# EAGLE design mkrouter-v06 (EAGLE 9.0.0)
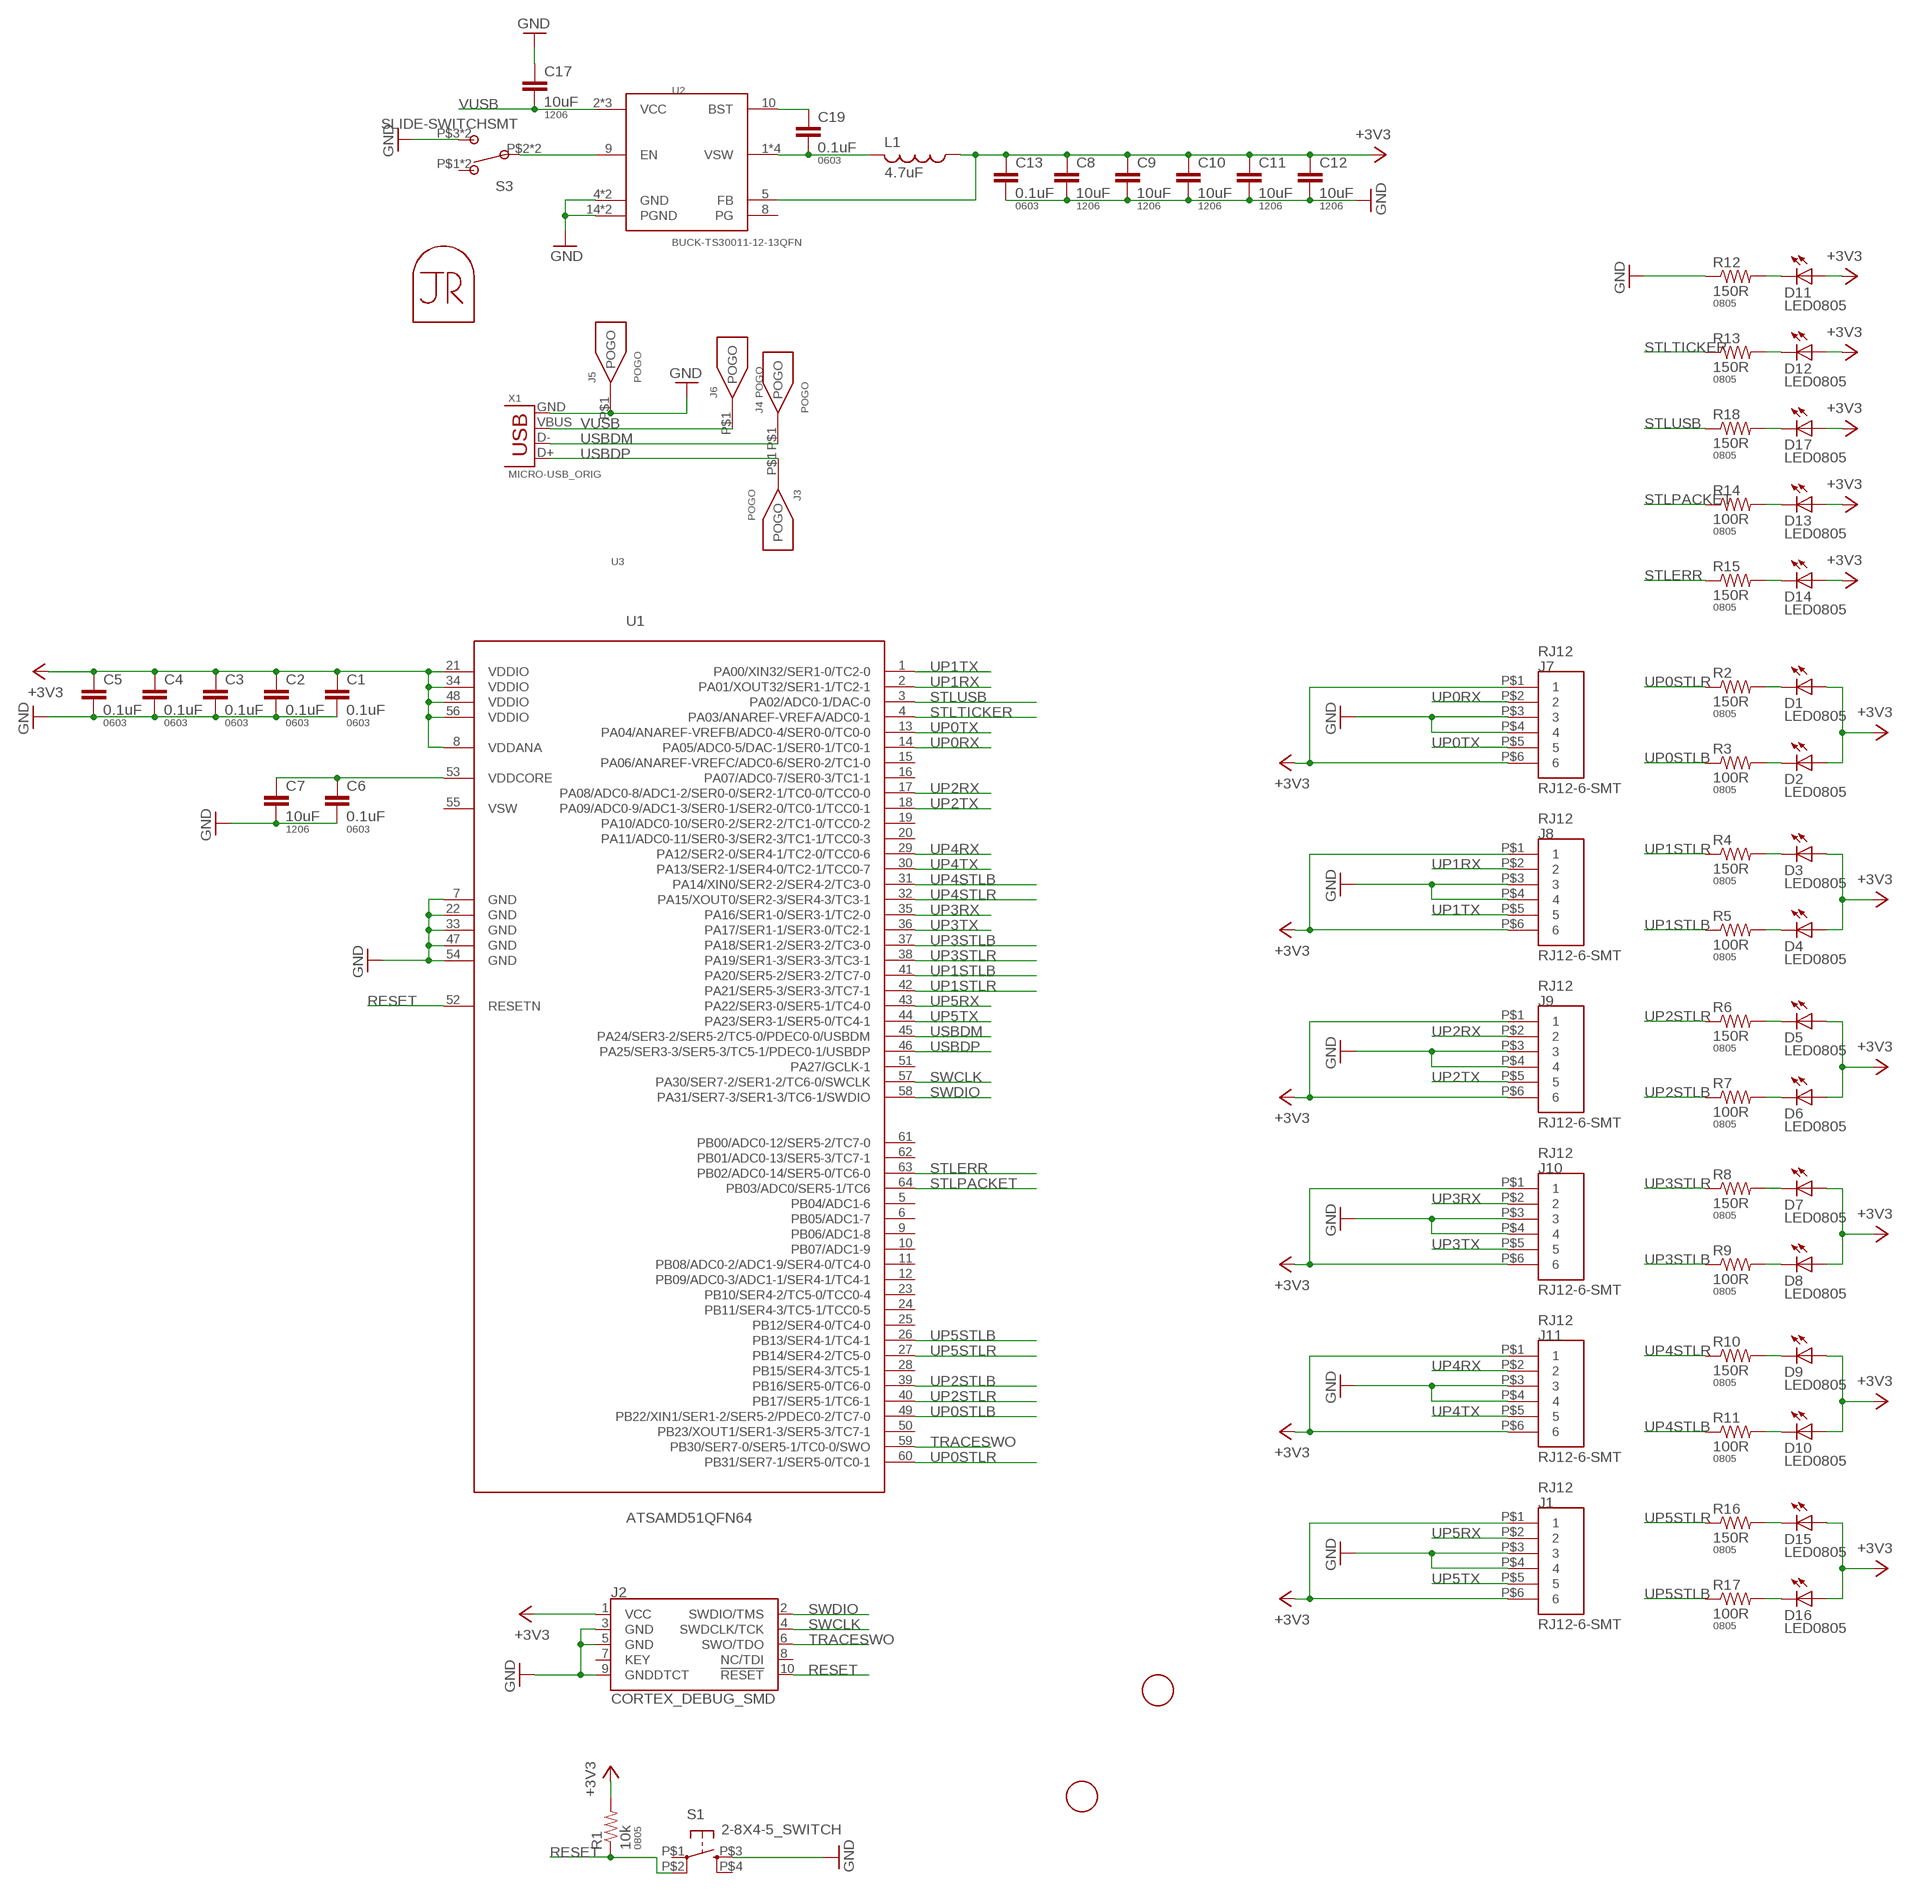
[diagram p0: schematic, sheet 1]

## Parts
C1  0.1uF  CAP0603-CAP  [0603-CAP]
C2  0.1uF  CAP0603-CAP  [0603-CAP]
C3  0.1uF  CAP0603-CAP  [0603-CAP]
C4  0.1uF  CAP0603-CAP  [0603-CAP]
C5  0.1uF  CAP0603-CAP  [0603-CAP]
C6  0.1uF  CAP0603-CAP  [0603-CAP]
C7  10uF  CAP1206  [1206]
C8  10uF  CAP1206  [1206]
C9  10uF  CAP1206  [1206]
C10  10uF  CAP1206  [1206]
C11  10uF  CAP1206  [1206]
C12  10uF  CAP1206  [1206]
C13  0.1uF  CAP0603-CAP  [0603-CAP]
C17  10uF  CAP1206  [1206]
C19  0.1uF  CAP0603-CAP  [0603-CAP]
D1  LED0805  [LED0805]
D2  LED0805  [LED0805]
D3  LED0805  [LED0805]
D4  LED0805  [LED0805]
D5  LED0805  [LED0805]
D6  LED0805  [LED0805]
D7  LED0805  [LED0805]
D8  LED0805  [LED0805]
D9  LED0805  [LED0805]
D10  LED0805  [LED0805]
D11  LED0805  [LED0805]
D12  LED0805  [LED0805]
D13  LED0805  [LED0805]
D14  LED0805  [LED0805]
D15  LED0805  [LED0805]
D16  LED0805  [LED0805]
D17  LED0805  [LED0805]
J1  RJ12-6-SMT  [RJ12-6-SMT]
J2  CORTEX_DEBUG_SMD  [SAMTECH_FTSH-105-01]
J3  POGO  [POGO]
J4  POGO  [POGO]
J5  POGO  [POGO]
J6  POGO  [POGO]
J7  RJ12-6-SMT  [RJ12-6-SMT]
J8  RJ12-6-SMT  [RJ12-6-SMT]
J9  RJ12-6-SMT  [RJ12-6-SMT]
J10  RJ12-6-SMT  [RJ12-6-SMT]
J11  RJ12-6-SMT  [RJ12-6-SMT]
L1  4.7uF  INDUCTOR  [NRS5020T4R7MMGJ]
MP1  JRTOMBSTONE  [JRTOMBSTONE]
R1  10k  RESISTOR0805-RES  [0805]
R2  150R  RESISTOR0805-RES  [0805]
R3  100R  RESISTOR0805-RES  [0805]
R4  150R  RESISTOR0805-RES  [0805]
R5  100R  RESISTOR0805-RES  [0805]
R6  150R  RESISTOR0805-RES  [0805]
R7  100R  RESISTOR0805-RES  [0805]
R8  150R  RESISTOR0805-RES  [0805]
R9  100R  RESISTOR0805-RES  [0805]
R10  150R  RESISTOR0805-RES  [0805]
R11  100R  RESISTOR0805-RES  [0805]
R12  150R  RESISTOR0805-RES  [0805]
R13  150R  RESISTOR0805-RES  [0805]
R14  100R  RESISTOR0805-RES  [0805]
R15  150R  RESISTOR0805-RES  [0805]
R16  150R  RESISTOR0805-RES  [0805]
R17  100R  RESISTOR0805-RES  [0805]
R18  150R  RESISTOR0805-RES  [0805]
S1  2-8X4-5_SWITCH  [TACT-SWITCH-KMR6]
S3  SLIDE-SWITCHSMT  [SLIDESWITCH-CL-SB-22A]
U1  ATSAMD51QFN64  [QFN-64-9X9MM]
U2  BUCK-TS30011-12-13QFN  [QFN16-3X3-TI-RTE]
U3  RASPBERRYPI-3BPLUS  [RASPBERRYPI-3BPLUS]
U$3  FIDUCIAL  [FIDUCIAL_1MM]
U$4  FIDUCIAL  [FIDUCIAL_1MM]
X1  MICRO-USB_ORIG  [DX4R005HJ5]

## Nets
+3V3: C1.1 C2.1 C3.1 C4.1 C5.1 C8.1 C9.1 C10.1 C11.1 C12.1 C13.1 D1.1(A) D2.1(A) D3.1(A) D4.1(A) D5.1(A) D6.1(A) D7.1(A) D8.1(A) D9.1(A) D10.1(A) D11.1(A) D12.1(A) D13.1(A) D14.1(A) D15.1(A) D16.1(A) D17.1(A) J1.P$1 J1.P$6 J2.1(VCC) J7.P$1 J7.P$6 J8.P$1 J8.P$6 J9.P$1 J9.P$6 J10.P$1 J10.P$6 J11.P$1 J11.P$6 L1.1 R1.2 U1.8(VDDANA) U1.21(VDDIO) U1.34(VDDIO) U1.48(VDDIO) U1.56(VDDIO) U2.5(FB)
BST: C19.1 U2.10(BST)
GND: C1.2 C2.2 C3.2 C4.2 C5.2 C6.2 C7.2 C8.2 C9.2 C10.2 C11.2 C12.2 C13.2 C17.1 J1.P$3 J1.P$4 J2.3(GND) J2.5(GND) J2.9(GNDDTCT) J5.P$1(POGO) J7.P$3 J7.P$4 J8.P$3 J8.P$4 J9.P$3 J9.P$4 J10.P$3 J10.P$4 J11.P$3 J11.P$4 R12.1 S1.P$3(S) S3.P$3 S3.P$6 U1.7(GND) U1.22(GND) U1.33(GND) U1.47(GND) U1.54(GND) U2.4(GND) U2.14(PGND) U2.15(PGND) U2.TH(GND) X1.GND
N$1: S3.P$2 S3.P$5 U2.9(EN)
N$2: D4.2(C) R5.2
N$3: D16.2(C) R17.2
N$4: D17.2(C) R18.2
N$5: D15.2(C) R16.2
N$6: D2.2(C) R3.2
N$8: D1.2(C) R2.2
N$9: D3.2(C) R4.2
N$10: D6.2(C) R7.2
N$11: D5.2(C) R6.2
N$12: D8.2(C) R9.2
N$13: D7.2(C) R8.2
N$14: D10.2(C) R11.2
N$15: D9.2(C) R10.2
N$16: D13.2(C) R14.2
N$17: D14.2(C) R15.2
N$22: D12.2(C) R13.2
N$23: D11.2(C) R12.2
RESET: J2.10(!RESET) R1.1 S1.P$2(P1) U1.52(RESETN)
STLERR: R15.1 U1.63(PB02/ADC0-14/SER5-0/TC6-0)
STLPACKET: R14.1 U1.64(PB03/ADC0/SER5-1/TC6)
STLTICKER: R13.1 U1.4(PA03/ANAREF-VREFA/ADC0-1)
STLUSB: R18.1 U1.3(PA02/ADC0-1/DAC-0)
SWCLK: J2.4(SWDCLK/TCK) U1.57(PA30/SER7-2/SER1-2/TC6-0/SWCLK)
SWDIO: J2.2(SWDIO/TMS) U1.58(PA31/SER7-3/SER1-3/TC6-1/SWDIO)
TRACESWO: J2.6(SWO/TDO) U1.59(PB30/SER7-0/SER5-1/TC0-0/SWO)
UP0RX: J7.P$2 U1.14(PA05/ADC0-5/DAC-1/SER0-1/TC0-1)
UP0STLB: R3.1 U1.49(PB22/XIN1/SER1-2/SER5-2/PDEC0-2/TC7-0)
UP0STLR: R2.1 U1.60(PB31/SER7-1/SER5-0/TC0-1)
UP0TX: J7.P$5 U1.13(PA04/ANAREF-VREFB/ADC0-4/SER0-0/TC0-0)
UP1RX: J8.P$2 U1.2(PA01/XOUT32/SER1-1/TC2-1)
UP1STLB: R5.1 U1.41(PA20/SER5-2/SER3-2/TC7-0)
UP1STLR: R4.1 U1.42(PA21/SER5-3/SER3-3/TC7-1)
UP1TX: J8.P$5 U1.1(PA00/XIN32/SER1-0/TC2-0)
UP2RX: J9.P$2 U1.17(PA08/ADC0-8/ADC1-2/SER0-0/SER2-1/TC0-0/TCC0-0)
UP2STLB: R7.1 U1.39(PB16/SER5-0/TC6-0)
UP2STLR: R6.1 U1.40(PB17/SER5-1/TC6-1)
UP2TX: J9.P$5 U1.18(PA09/ADC0-9/ADC1-3/SER0-1/SER2-0/TC0-1/TCC0-1)
UP3RX: J10.P$2 U1.35(PA16/SER1-0/SER3-1/TC2-0)
UP3STLB: R9.1 U1.37(PA18/SER1-2/SER3-2/TC3-0)
UP3STLR: R8.1 U1.38(PA19/SER1-3/SER3-3/TC3-1)
UP3TX: J10.P$5 U1.36(PA17/SER1-1/SER3-0/TC2-1)
UP4RX: J11.P$2 U1.29(PA12/SER2-0/SER4-1/TC2-0/TCC0-6)
UP4STLB: R11.1 U1.31(PA14/XIN0/SER2-2/SER4-2/TC3-0)
UP4STLR: R10.1 U1.32(PA15/XOUT0/SER2-3/SER4-3/TC3-1)
UP4TX: J11.P$5 U1.30(PA13/SER2-1/SER4-0/TC2-1/TCC0-7)
UP5RX: J1.P$2 U1.43(PA22/SER3-0/SER5-1/TC4-0)
UP5STLB: R17.1 U1.26(PB13/SER4-1/TC4-1)
UP5STLR: R16.1 U1.27(PB14/SER4-2/TC5-0)
UP5TX: J1.P$5 U1.44(PA23/SER3-1/SER5-0/TC4-1)
USBDM: J4.P$1(POGO) U1.45(PA24/SER3-2/SER5-2/TC5-0/PDEC0-0/USBDM) X1.D-
USBDP: J3.P$1(POGO) U1.46(PA25/SER3-3/SER5-3/TC5-1/PDEC0-1/USBDP) X1.D+
VDDCORE: C6.1 C7.1 U1.53(VDDCORE)
VSW: C19.2 L1.2 U2.1(VSW) U2.12(VSW) U2.13(VSW) U2.16(VSW)
VUSB: C17.2 J6.P$1(POGO) U2.2(VCC) U2.3(VCC) U2.11(VCC) X1.VBUS
Unconnected: J2.7(KEY) J2.8(NC/TDI) S1.P$1(P) S1.P$4(S1) S3.P$1 S3.P$4 U1.5(PB04/ADC1-6) U1.6(PB05/ADC1-7) U1.9(PB06/ADC1-8) U1.10(PB07/ADC1-9) U1.11(PB08/ADC0-2/ADC1-9/SER4-0/TC4-0) U1.12(PB09/ADC0-3/ADC1-1/SER4-1/TC4-1) U1.15(PA06/ANAREF-VREFC/ADC0-6/SER0-2/TC1-0) U1.16(PA07/ADC0-7/SER0-3/TC1-1) U1.19(PA10/ADC0-10/SER0-2/SER2-2/TC1-0/TCC0-2) U1.20(PA11/ADC0-11/SER0-3/SER2-3/TC1-1/TCC0-3) U1.23(PB10/SER4-2/TC5-0/TCC0-4) U1.24(PB11/SER4-3/TC5-1/TCC0-5) U1.25(PB12/SER4-0/TC4-0) U1.28(PB15/SER4-3/TC5-1) U1.50(PB23/XOUT1/SER1-3/SER5-3/TC7-1) U1.51(PA27/GCLK-1) U1.55(VSW) U1.61(PB00/ADC0-12/SER5-2/TC7-0) U1.62(PB01/ADC0-13/SER5-3/TC7-1) U2.8(PG)

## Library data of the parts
C1-C6 C13 C19 = borkedlabs-passives:CAP: Capacitor; PACKAGE: 0603
C7-C12 C17 = borkedlabs-passives:CAP: Capacitor; PACKAGE: 1206
D1-D17 = lights:LED: LED
J1 J7-J11 = connector:RJ12-6-SMT
J2 = SparkFun-Connectors:CORTEX_DEBUG: Cortex Debug Connector - 10 pin Supports JTAG debug, Serial Wire debug, and Serial Wire Viewer. PTH and SMD connector options available. General Connector Information Products: PTH Connector -via Digi-Key SparkFun PSoc SparkFun T
J3-J6 = connector:POGO
L1 = power:INDUCTOR
MP1 = connector:JRTOMBSTONE
R1-R18 = borkedlabs-passives:RESISTOR: Resistor; PACKAGE: 0805
S1 = fab:2-8X4-5_SWITCH
S3 = fab:SLIDE-SWITCH: SMD slide-switch AYZ0102AGRLC as found in the fablab inventory. Includes the mounting holes. Made by Zaerc.
U1 = microcontrollers:ATSAMD51
U2 = power:BUCK-TS30011-12-13
U3 = connector:RASPBERRYPI-3BPLUS
U$3 U$4 = borkedlabs-misc:FIDUCIAL: For use by pick and place machines to calibrate the vision/machine, 1mm
X1 = fab:MICRO-USB: SMD micro USB connector as found in the fablab inventory. Three footprint variants included: original, as described by manufacturer's datasheet for milling with the 1/100" bit for milling with the 1/64" bit Made by Zaerc.

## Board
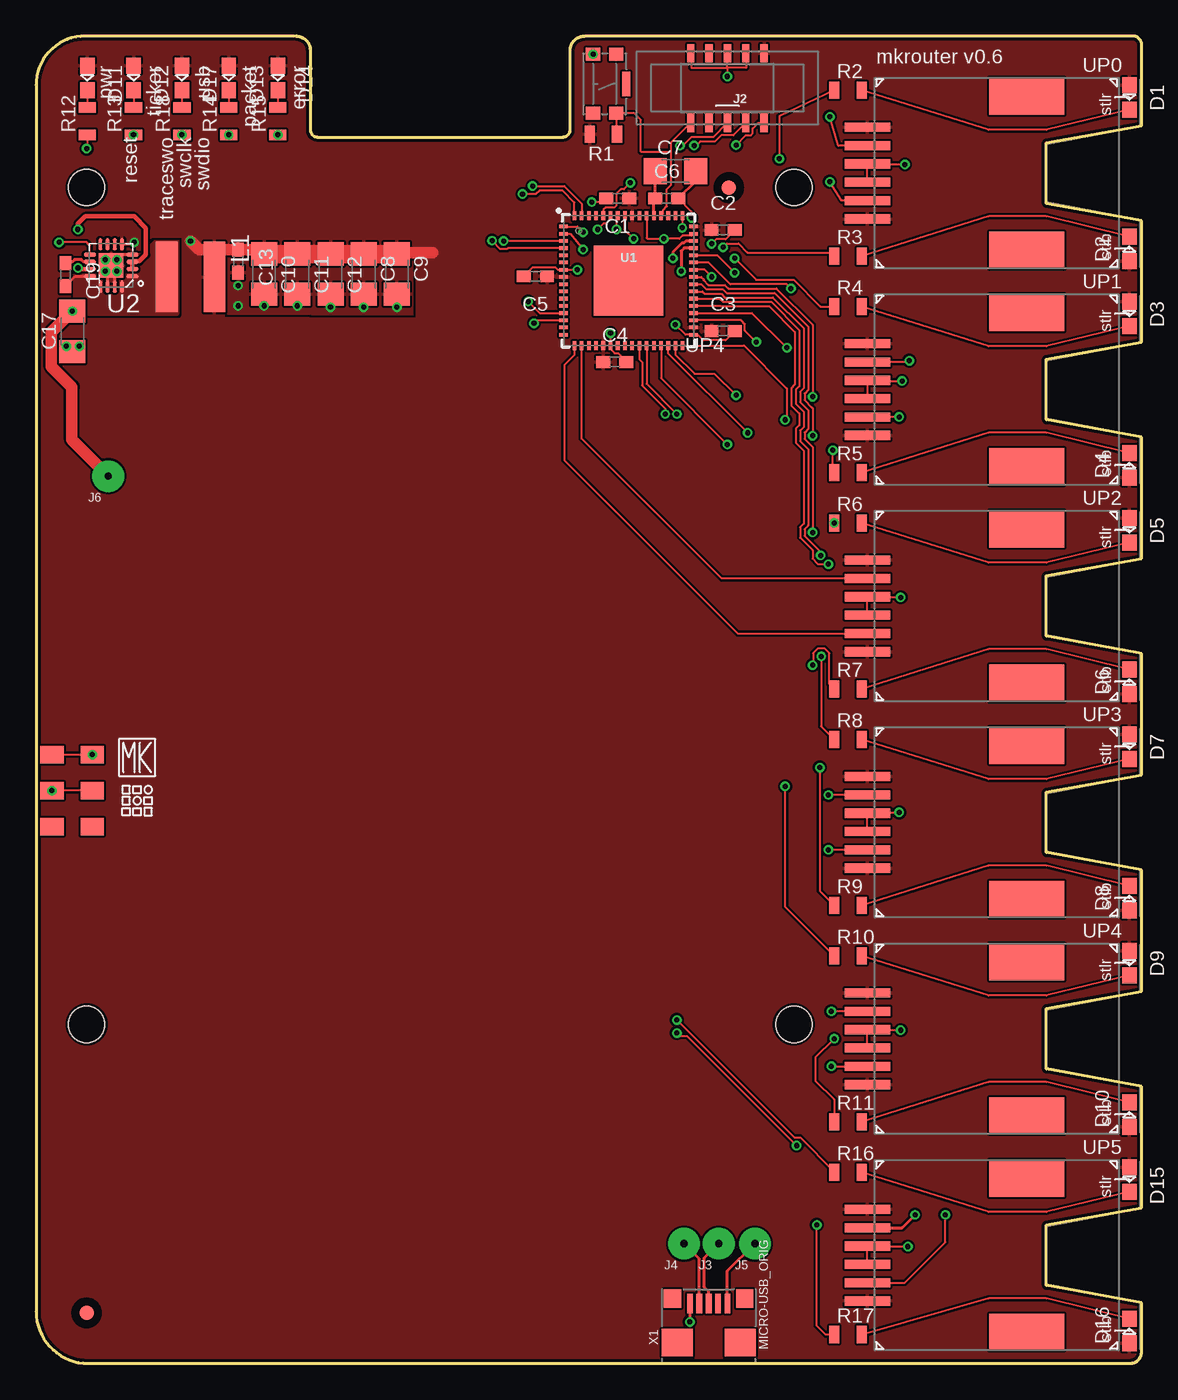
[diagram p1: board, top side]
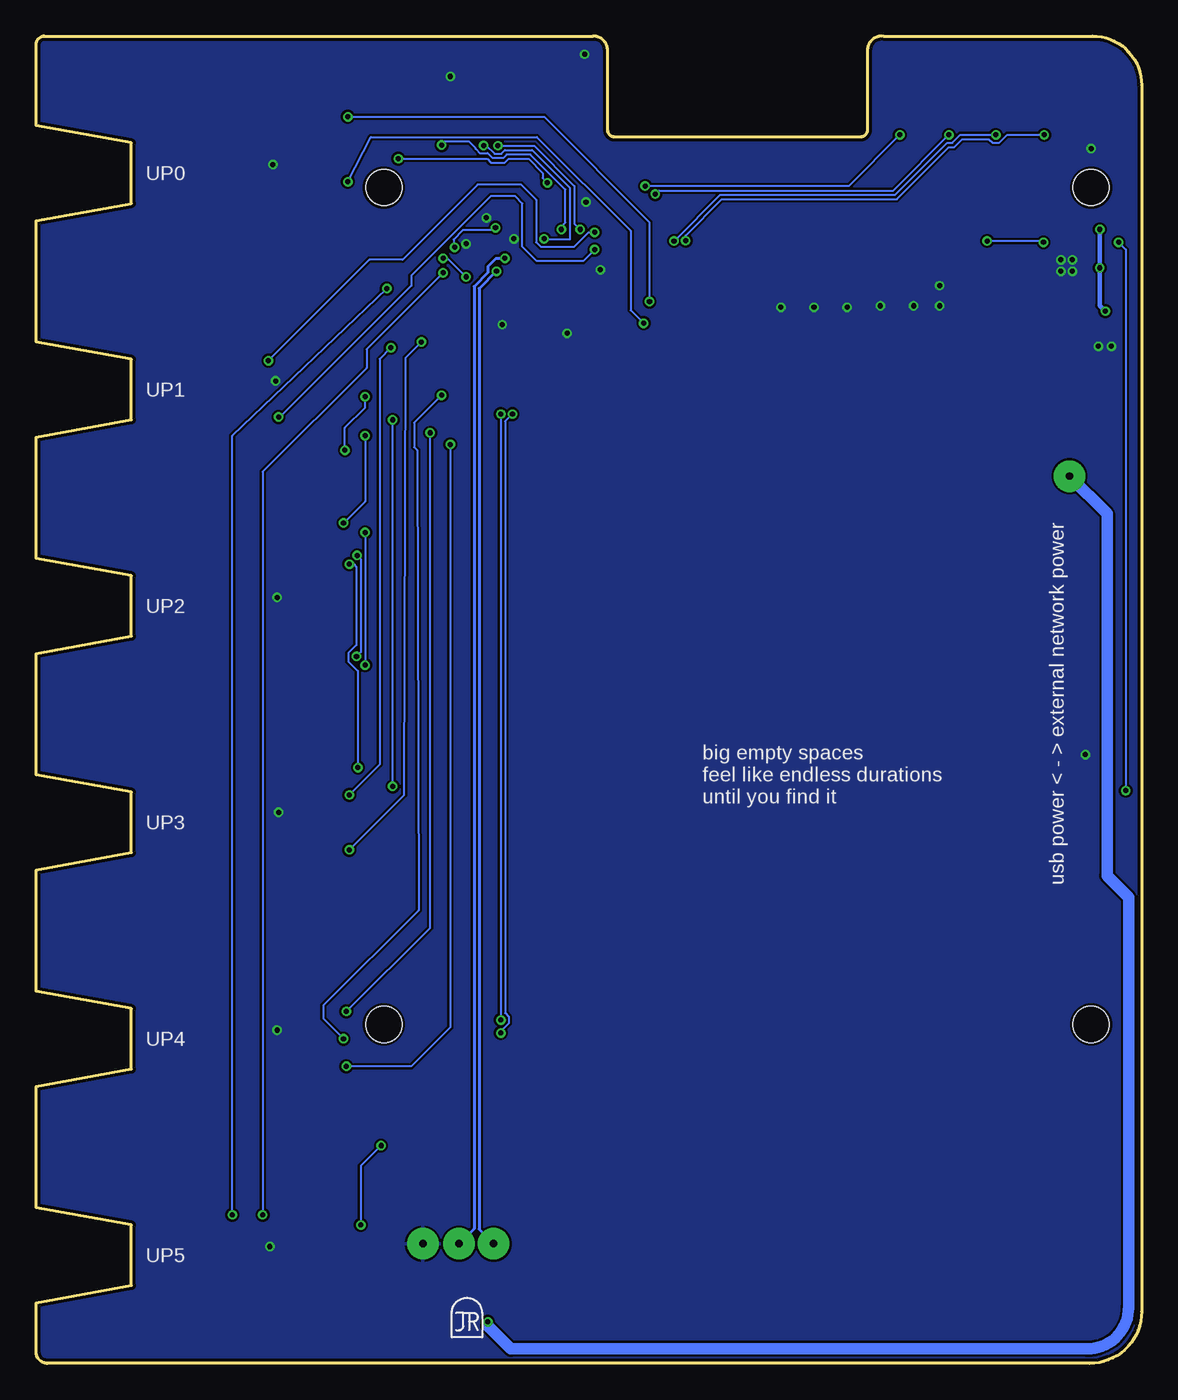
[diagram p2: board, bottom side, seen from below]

Size 76.6 x 92 mm. Coordinates in mm from the lower left corner, seen from the top.
Outline: 17.9,92 3.4,92 arc90 0,88.6 0,3.6 arc90 3.6,0 75.8,0 arc90 76.6,0.8 76.6,4.2 70,5.4 70,9.6 76.6,10.8 76.6,19.2 70,20.4 70,24.6 76.6,25.8 76.6,34.2 70,35.4 70,39.6 76.6,40.8 76.6,49.2 70,50.4 70,54.6 76.6,55.8 76.6,64.2 70,65.4 70,69.6 76.6,70.8 76.6,79.2 70,80.4 70,84.6 76.6,85.8 76.6,91.4 arc90 76,92 38,92 arc90 37,91 37,85.5 arc-90 36.5,85 19.5,85 arc-90 19,85.5 19,91 arc90 18,92
Copper layers (1*16): Top 0.035mm / dielectric 1.5mm / Bottom 0.035mm
Design rules "default *": minimum track width 6mil, minimum drill 0.3mm, track to track 6mil, track to pad 6mil, pad to pad 6mil, via to via 6mil, smd to smd 6mil, copper to edge 8mil, drill to drill 8mil, minimum pad ring 10mil, minimum via ring 6mil, stop-mask expansion 4mil, vias tented up to drill 20mil, thermal gap 6mil

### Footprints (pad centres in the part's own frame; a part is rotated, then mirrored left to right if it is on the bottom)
0603-CAP = smd 0.96 x 0.8: 1 -0.8,0; 2 0.8,0
1206 = smd 1.6 x 1.8: 1 -1.4,0; 2 1.4,0
LED0805 = smd 1.1 x 1: 1 -0.85,0; 2 0.85,0
RJ12-6-SMT = smd 0.635 x 3.175: P$1 -3.175,17.399; P$2 -1.905,17.399; P$3 -0.635,17.399; P$4 0.635,17.399; P$5 1.905,17.399; P$6 3.175,17.399 | smd 2.54 x 5.207: P$7 -5.334,6.35; P$8 5.334,6.35
SAMTECH_FTSH-105-01 = smd 0.508 x 1.27: 1 -2.54,-2.413; 2 -2.54,2.413; 3 -1.27,-2.413; 4 -1.27,2.413; 5 0,-2.413; 6 0,2.413; 7 1.27,-2.413; 8 1.27,2.413; 9 2.54,-2.413; 10 2.54,2.413
POGO = drill 0.51 pad 2.184: P$1 0,0
NRS5020T4R7MMGJ = smd 4.9 x 1.5: 1 0,1.65; 2 0,-1.65
0805 = smd 0.7 x 1.2: 1 -0.95,0; 2 0.95,0
TACT-SWITCH-KMR6 = smd 0.9 x 1: P$1 -2.05,0.8; P$2 2.05,0.8; P$3 -2.05,-0.8; P$4 2.05,-0.8 | smd 1.7 x 0.55: P$5 0,1.5
SLIDESWITCH-CL-SB-22A = smd 1.2 x 1.6: P$1 -2.5,1.4; P$2 0,1.4; P$3 2.5,1.4; P$4 -2.5,-1.4; P$5 0,-1.4; P$6 2.5,-1.4
QFN-64-9X9MM = smd 0.6 x 0.25: 1 -4.5,3.75; 2 -4.5,3.25; 3 -4.5,2.75; 4 -4.5,2.25; 5 -4.5,1.75; 6 -4.5,1.25; 7 -4.5,0.75; 8 -4.5,0.25; 9 -4.5,-0.25; 10 -4.5,-0.75; 11 -4.5,-1.25; 12 -4.5,-1.75; 13 -4.5,-2.25; 14 -4.5,-2.75; 15 -4.5,-3.25; 16 -4.5,-3.75; 33 4.5,-3.75; 34 4.5,-3.25; 35 4.5,-2.75; 36 4.5,-2.25; 37 4.5,-1.75; 38 4.5,-1.25; 39 4.5,-0.75; 40 4.5,-0.25; 41 4.5,0.25; 42 4.5,0.75; 43 4.5,1.25; 44 4.5,1.75; 45 4.5,2.25; 46 4.5,2.75; 47 4.5,3.25; 48 4.5,3.75 | smd 0.25 x 0.6: 17 -3.75,-4.5; 18 -3.25,-4.5; 19 -2.75,-4.5; 20 -2.25,-4.5; 21 -1.75,-4.5; 22 -1.25,-4.5; 23 -0.75,-4.5; 24 -0.25,-4.5; 25 0.25,-4.5; 26 0.75,-4.5; 27 1.25,-4.5; 28 1.75,-4.5; 29 2.25,-4.5; 30 2.75,-4.5; 31 3.25,-4.5; 32 3.75,-4.5; 49 3.75,4.5; 50 3.25,4.5; 51 2.75,4.5; 52 2.25,4.5; 53 1.75,4.5; 54 1.25,4.5; 55 0.75,4.5; 56 0.25,4.5; 57 -0.25,4.5; 58 -0.75,4.5; 59 -1.25,4.5; 60 -1.75,4.5; 61 -2.25,4.5; 62 -2.75,4.5; 63 -3.25,4.5; 64 -3.75,4.5 | smd 4.826 x 4.826: P$1 0,0
QFN16-3X3-TI-RTE = smd 0.85 x 0.3: 1 -1.475,0.75; 2 -1.475,0.25; 3 -1.475,-0.25; 4 -1.475,-0.75; 9 1.475,-0.75; 10 1.475,-0.25; 11 1.475,0.25; 12 1.475,0.75 | smd 0.3 x 0.85: 5 -0.75,-1.475; 6 -0.25,-1.475; 7 0.25,-1.475; 8 0.75,-1.475; 13 0.75,1.475; 14 0.25,1.475; 15 -0.25,1.475; 16 -0.75,1.475 | smd 1.7 x 1.7: TH 0,0
RASPBERRYPI-3BPLUS = hole 2.5: 52.5,81.5; 3.5,81.5; 3.5,23.5; 52.5,23.5
FIDUCIAL_1MM = smd 1 x 1: 1 0,0
DX4R005HJ5 = smd 0.4 x 1.35: D+ 0,1.6; D- -0.65,1.6; GND 1.3,1.6; ID 0.65,1.6; VBUS -1.3,1.6 | smd 1.2 x 1.3: GND@1 -2.5,1.95; GND@2 2.5,1.95 | smd 2.15 x 1.9: GND@3 -2.175,-1.1; GND@4 2.175,-1.1

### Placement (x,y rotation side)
C1  40.3,80.75 180 top
C2  47.6,78.55 0 top
C3  47.6,71.55 0 top
C4  40.1,69.4 0 top
C5  34.6,75.35 180 top
C6  43.7,80.75 0 top
C7  44.3,82.65 0 top
C8  22.7,75.5 270 top
C9  25,75.5 270 top
C10  15.8,75.5 270 top
C11  18.1,75.5 270 top
C12  20.4,75.5 270 top
C13  14,76.4 270 top
C17  2.52,71.54 90 top
C19  2.02,75.46 270 top
D1  75.75,87.75 270 top
D2  75.75,77.25 90 top
D3  75.75,72.75 270 top
D4  75.75,62.25 90 top
D5  75.75,57.75 270 top
D6  75.75,47.25 90 top
D7  75.75,42.75 270 top
D8  75.75,32.25 90 top
D9  75.75,27.75 270 top
D10  75.75,17.25 90 top
D11  3.55,89.1 270 top
D12  6.75,89.1 270 top
D13  13.35,89.1 270 top
D14  16.75,89.1 270 top
D15  75.75,12.75 270 top
D16  75.75,2.25 90 top
D17  10.1,89.1 270 top
J1  75,7.5 90 top
J2  47.9,88.4 180 top
J3  47.3,8.3 0 top
J4  44.9,8.3 0 top
J5  49.8,8.3 0 top
J6  5,61.5 0 top
J7  75,82.5 90 top
J8  75,67.5 90 top
J9  75,52.5 90 top
J10  75,37.5 90 top
J11  75,22.5 90 top
L1  10.7,75.3 270 top
MP1  46.7,2.8 0 bottom
R1  39.3,85.2 180 top
R2  56.25,88.25 0 top
R3  56.25,76.75 0 top
R4  56.25,73.25 0 top
R5  56.25,61.75 0 top
R6  56.25,58.25 0 top
R7  56.25,46.75 0 top
R8  56.25,43.25 0 top
R9  56.25,31.75 0 top
R10  56.25,28.25 0 top
R11  56.25,16.75 0 top
R12  3.55,86.1 90 top
R13  6.75,86.1 90 top
R14  13.35,86.1 90 top
R15  16.75,86.1 90 top
R16  56.25,13.25 0 top
R17  56.25,2 0 top
R18  10.1,86.1 90 top
S1  39.4,88.69 270 top
S3  2.5,39.7 90 top
U1  41.05,75.05 0 top
U2  5.2,76.1 180 top
U3  0,0 0 top
U$1  [CBA-SILK-LOGO]  7,39 270 top
U$2  [MK-LOGO-SILK]  7,42 0 top
U$3  3.5,3.5 0 top
U$4  48,81.5 0 top
X1  46.6,2.55 0 top

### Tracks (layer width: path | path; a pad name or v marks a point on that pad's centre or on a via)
+3V3  (via drill 0.35)
  Top 0.152: U2.5 6.67,77.58 v6.8,77.7
  Top 0.813: C10.1 15.5,77.2 C13.1 12.8,77.2 | 12.8,77.2 12.3,76.7 12.35,76.65 L1.1 | v10.7,77.8 11.3,77.2 12.8,77.2 | C9.1 25.1,77 27.5,77
  Top 1.27: C10.1 C11.1 C12.1 C8.1 C9.1
  Bottom 0.152: v6.8,77.7 6.9,77.8 v10.7,77.8
  pour Top (rank 6): -1,94 78,94 78,-1 -1,-1
BST
  Top 0.203: C19.1 2.12,76.35 2.5,76.35 2.66,76.51 3.15,76.51 3.31,76.35 U2.10
GND  (via drill 0.35)
  Top 0.152: v37.5,75.8 U1.7 36.15,75.8 35.98,75.98 34.43,75.98 C5.2 | J2.9 45.4,90.77 45.4,89.8 47.9,89.8 | 47.9,89.8 J2.5 | J2.3 49.2,90.78 49.2,89.8 47.9,89.8 | 47.9,89.8 v47.9,89.2 | C4.2 40.9,69.45 40.33,70.02 40.08,70.02 39.8,70.3 U1.22 v39.8,71.4 | v44.3,72 45,71.3 U1.33 45.85,71.3 46.23,70.92 47.77,70.92 C3.2 | J8.P$3 J8.P$4 57.64,68.1 v60,68.1 | J7.P$3 J7.P$4 60.16,83.14 v60.2,83.1 | J9.P$3 J9.P$4 59.87,53.13 v59.9,53.1 | J10.P$3 J10.P$4 57.67,38.2 v59.8,38.2 | J11.P$3 J11.P$4 59.87,23.14 v59.9,23.1 | J1.P$3 J1.P$4 60.37,8.13 v60.4,8.1 | C1.2 39.25,80.5 v38.5,80.5 | C6.2 45.41,79.84 v45.41,79.41 | R12.1 3.55,84.25 v3.5,84.2 | S3.P$3 S3.P$6 | U1.54 42.3,78 42.36,77.94 v43.5,77.94 44.57,77.94 44.78,78.15 45.4,78.15 U1.47 | C2.2 47.77,77.92 47.12,77.92 v46.8,77.6
  Top 0.203: X1.GND 47.9,6.4 J5.P$1 | C7.2 45.7,81.95 C6.2 | 6.7,76.88 U2.4 5.95,76.85 v5.6,76.5 | U2.15 5.45,75.55 v5.6,75.7 | U2.14 4.95,75.55 v4.8,75.7 | v3,70.5 2.64,70.14 C17.1 2.15,70.5 v2.1,70.5
  other vias: 38.6,90.74 4.8,76.5 14,73.3 15.8,73.3 18.1,73.3 20.4,73.2 22.7,73.2 25,73.2 14,74.7 3.9,42.2
  pour Bottom: -2,95 79,95 79,-2 -2,-2
  pour Top (rank 2): 5.1,78.2 5.1,72.8 26.1,72.7 26.1,78.2
N$1  (via drill 0.35)
  Top 0.152: U2.9 3.73,77.47 3.5,77.7 v1.6,77.7 | S3.P$5 S3.P$2
  Bottom 0.152: v1.6,77.7 1.1,77.2 S3.P$2
  other vias: 1.1,39.7
N$2
  Top 0.152: D4.2 70,64.5 66,64.5 R5.2
N$3
  Top 0.152: D16.2 70,4.5 66,4.5 R17.2
N$4
  Top 0.152: D17.2 R18.2
N$5
  Top 0.152: D15.2 70,10.5 66,10.5 R16.2
N$6
  Top 0.152: D2.2 70,79.5 66,79.5 R3.2
N$8
  Top 0.152: D1.2 70,85.5 66,85.5 R2.2
N$9
  Top 0.152: D3.2 70,70.5 66,70.5 R4.2
N$10
  Top 0.152: D6.2 70,49.5 66,49.5 R7.2
N$11
  Top 0.152: D5.2 70,55.5 66,55.5 R6.2
N$12
  Top 0.152: D8.2 70,34.5 66,34.5 R9.2
N$13
  Top 0.152: D7.2 70,40.5 66,40.5 R8.2
N$14
  Top 0.152: D10.2 70,19.5 66,19.5 R11.2
N$15
  Top 0.152: D9.2 70,25.5 66,25.5 R10.2
N$16
  Top 0.152: D13.2 R14.2
N$17
  Top 0.152: D14.2 R15.2
N$22
  Top 0.152: D12.2 R13.2
N$23
  Top 0.152: D11.2 R12.2
RESET
  Top 0.152: U1.52 43.45,79.7 43.45,79.94 43.7,80.2 43.7,81.4 44,81.7 44,84 | J2.10 44,84.63 44,84 | 44,84 41.9,84 41.9,86.2 41.46,86.64 S1.P$2 40.2,85.25 R1.1
STLERR  (via drill 0.35)
  Top 0.152: v34.4,81.6 36.6,81.6 37.8,80.4 U1.63
  Bottom 0.152: R15.1 20.3,81.6 v34.4,81.6
  other vias: 16.75,85.15
STLPACKET  (via drill 0.35)
  Top 0.152: U1.64 37.3,80.47 36.47,81.3 34.88,81.3 34.63,81.04 v33.7,81.04
  Bottom 0.152: v33.7,81.04 33.45,81.3 17.2,81.3 R14.1
  other vias: 13.35,85.15
STLTICKER  (via drill 0.35)
  Top 0.152: U1.4 32.69,77.3 32.63,77.24 32.17,77.24 v31.59,77.82
  Bottom 0.152: v31.59,77.82 31.59,78.18 29.08,80.69 16.95,80.69 13.35,84.29 12.99,84.29 12.44,84.84 10.58,84.84 10.33,84.59 9.87,84.59 9.31,85.15 R13.1
  other vias: 6.75,85.15
STLUSB  (via drill 0.35)
  Top 0.152: U1.3 v32.4,77.8
  Bottom 0.152: v32.4,77.8 29.21,80.99 17.08,80.99 13.47,84.59 13.12,84.59 12.56,85.15 R18.1
  other vias: 10.1,85.15
SWCLK  (via drill 0.35)
  Top 0.152: J2.4 48.31,85.12 47.47,85.12 47.04,84.69 46,84.69 45.71,84.41 v45.59,84.41 | v41.4,77.94 40.8,78.54 U1.57
  Bottom 0.152: v45.59,84.41 45.39,84.41 44.83,83.84 44.37,83.84 44.12,84.09 42.23,84.09 39.62,81.48 39.62,77.92 39.6,77.9 41.36,77.9 v41.4,77.94
SWDIO  (via drill 0.35)
  Top 0.152: U1.58 40.2,79.45 v40.2,78.6 | J2.2 50.04,85.99 49.65,85.6 49.65,85.26 49.52,85.12 49.18,85.12 v48.5,84.44
  Bottom 0.152: v40.2,78.6 40.2,78.8 39.92,79.08 39.92,81.36 42.35,83.79 43.99,83.79 44.24,83.54 44.96,83.54 45.32,83.9 45.36,83.85 45.82,83.85 46.15,84.18 46.15,84.24 46.6,84.69 48.3,84.69 48.3,84.64 v48.5,84.44
TRACESWO  (via drill 0.35)
  Top 0.152: J2.6 46.91,85 45.4,85 44.8,84.4 v44.6,84.4 | v38.9,78.6 39.32,79.02 39.52,79.02 39.8,79.3 U1.59
  Bottom 0.152: v44.6,84.4 42.1,84.4 39.3,81.6 39.3,79 v38.9,78.6
UP0RX  (via drill 0.35)
  Top 0.152: J7.P$2 55.8,80.59 v55,81.9 | v34.5,72.1 34.7,72.3 U1.14
  Bottom 0.152: v55,81.9 53.4,85 41.9,85 35.4,78.5 35.4,73 v34.5,72.1
UP0STLB  (via drill 0.35)
  Top 0.152: v47.61,77.36 47.86,77.62 48.67,77.62 49.29,77 55.05,77 R3.1 | U1.49 44.77,79.52 v44.77,78.71
  Bottom 0.152: v47.61,77.36 47.68,77.43 47.68,77.89 47.04,78.53 44.95,78.53 v44.77,78.71
UP0STLR  (via drill 0.35)
  Top 0.152: R2.1 51.5,86.45 v51.5,83.5 | U1.60 39.3,79.95 39.47,80.12 40.08,80.12 40.21,80.25 40.21,81.06 40.52,81.38 40.73,81.38 v41.17,81.83
  Bottom 0.152: v51.5,83.5 45.35,83.5 45.08,83.23 44.12,83.23 43.87,83.49 42.48,83.49 41.5,82.51 41.5,82.15 v41.17,81.83
UP0TX  (via drill 0.35)
  Top 0.152: J7.P$5 55.6,84.4 v55,86.4 | v34.1,73.6 34.9,72.8 U1.13
  Bottom 0.152: v55,86.4 41.4,86.4 34.1,79.1 v34.1,73.6
UP1RX  (via drill 0.35)
  Top 0.152: U1.2 37,78.3 v37.9,77.2 | v59.8,65.6 J8.P$2
  Bottom 0.152: v37.9,77.2 38.7,76.4 41.9,76.4 42.9,77.4 42.9,80.4 43.4,80.9 45.1,80.9 50.6,75.4 50.6,74.7 59.7,65.6 v59.8,65.6
UP1STLB  (via drill 0.35)
  Top 0.152: U1.41 46.1,75.3 46.25,75.15 46.25,75.08 46.58,74.75 47.72,74.75 47.97,74.5 51.3,74.5 53.8,72 v53.8,67 | R5.1 55.2,61.85 v55.2,63.3
  Bottom 0.152: v53.8,67 53.8,66.25 55.2,64.85 v55.2,63.3
UP1STLR  (via drill 0.35)
  Top 0.152: v46.81,75.31 46.31,75.8 U1.42 | R4.1 54.34,73.25 52.48,75.11 49.9,75.11 v48.4,76.6
  Bottom 0.152: v48.4,76.6 48.1,76.6 v46.81,75.31
UP1TX  (via drill 0.35)
  Top 0.152: v37.9,78.4 37.5,78.8 U1.1 | v60.5,69.5 60.41,69.41 J8.P$5
  Bottom 0.152: 38.1,78.4 v37.9,78.4 38.31,78.4 39.33,77.39 41.63,77.39 41.96,77.71 41.96,80.66 43,81.7 46,81.7 51.2,76.5 53.5,76.5 v60.5,69.5
UP2RX
  Top 0.152: U1.17 37.3,69.9 36.6,69.2 36.6,62.6 48.6,50.59 J9.P$2
UP2STLB  (via drill 0.35)
  Top 0.152: U1.39 46.16,74.3 46.32,74.14 47.47,74.14 47.72,73.89 51.05,73.89 53.19,71.74 53.19,67.61 52.94,67.36 52.94,66.64 53.49,66.09 53.49,64.78 53.24,64.53 53.24,64.07 53.8,63.51 v53.8,57.6 | v53.8,48.4 53.8,48.25 53.84,48.29 53.84,49.23 54.17,49.56 54.63,49.56 54.96,49.23 54.96,47.09 R7.1
  Bottom 0.152: v53.8,57.6 v53.8,48.4 53.8,48.25
UP2STLR  (via drill 0.35)
  Top 0.152: U1.40 46.1,74.8 46.45,74.45 47.59,74.45 47.85,74.19 51.17,74.19 53.49,71.87 53.49,67.48 53.24,67.23 53.24,66.77 53.76,66.26 53.8,66.21 v53.8,64.3
  Bottom 0.152: v53.8,64.3 53.8,59.75 R6.1
  other vias: 55.3,58.25
UP2TX
  Top 0.152: J9.P$5 47.49,54.41 37.8,64.1 U1.18
UP3RX  (via drill 0.35)
  Top 0.152: J10.P$2 v54.9,35.6 | v49.9,70.8 49.11,71.59 49.11,72.05 48.85,72.3 U1.35
  Bottom 0.152: v54.9,35.6 51.1,39.4 51,69.7 v49.9,70.8
UP3STLB  (via drill 0.35)
  Top 0.152: U1.37 47.45,73.3 47.47,73.28 50.8,73.28 52.58,71.49 52.58,67.86 52.33,67.61 52.33,66.39 52.89,65.83 52.89,65.03 52.63,64.78 52.63,63.82 53.19,63.26 53.19,58.21 52.94,57.96 52.94,57.23 53.8,56.37 53.8,55.77 54.17,55.4 v54.9,55.4 | v54.3,41.3 54.3,32.75 R9.1
  Bottom 0.152: v54.9,55.4 54.6,55.4 54.41,55.21 54.41,49.78 54.96,49.23 54.96,48.66 54.3,48 v54.3,41.3
UP3STLR  (via drill 0.35)
  Top 0.152: U1.38 47.38,73.8 47.59,73.58 50.92,73.58 52.89,71.62 52.89,67.73 52.63,67.48 52.63,66.52 53.19,65.96 53.19,64.91 52.94,64.66 52.94,63.94 53.49,63.39 53.49,58.08 53.24,57.83 53.24,57.36 54.36,56.24 v54.36,56 | v54.4,49 54.4,44.15 R8.1
  Bottom 0.152: v54.36,56 54.1,55.75 54.1,49.3 v54.4,49.01 v54.4,49
UP3TX  (via drill 0.35)
  Top 0.152: J10.P$5 v54.91,39.41 v54.9,39.4 | U1.36 49.6,72.8 52,70.4 v52.02,70.4
  Bottom 0.152: v54.9,39.4 52.8,41.5 52.8,69.62 v52.02,70.4
UP4RX  (via drill 0.35)
  Top 0.152: U1.29 43.3,68.3 v47.9,63.7 | v55.1,20.6 v55.1,20.59 J11.P$2
  Bottom 0.152: v55.1,20.6 50.6,20.6 47.9,23.3 v47.9,63.7
UP4STLB  (via drill 0.35)
  Top 0.152: U1.31 44.3,69.93 45.63,68.6 47,68.6 v48.5,67.1 | v55.3,22.5 54,21.2 54,19.6 55.3,18.3 R11.1
  Bottom 0.152: v48.5,67.1 50.4,65.2 50.4,63.5 50.2,63.3 50.1,31.4 56.7,24.8 56.7,23.9 v55.3,22.5
UP4STLR  (via drill 0.35)
  Top 0.152: R10.1 51.9,31.65 v51.9,40 | U1.32 49.05,70.55 52.02,67.58 52.02,65.53 v51.9,65.4
  Bottom 0.152: v51.9,40 v51.9,65.4
UP4TX  (via drill 0.35)
  Top 0.152: J11.P$5 v55.1,24.41 v55.1,24.4 | v49.3,64.5 43.8,70 U1.30
  Bottom 0.152: v55.1,24.4 49.3,30.2 v49.3,64.5
UP5RX  (via drill 0.35)
  Top 0.152: J1.P$2 60.2,5.59 63,8.4 v63,10.3 | v52.3,74.5 52,74.8 48.1,74.8 46.6,76.3 U1.43
  Bottom 0.152: v63,10.3 63,64.3 v52.3,74.5
UP5STLB  (via drill 0.35)
  Top 0.152: U1.26 41.8,69.6 41.99,69.41 41.99,67.77 43.59,66.18 v43.59,65.8 | v44.4,22.9 44.6,22.7 45.07,22.7 52.67,15.1 v52.7,15.1 | R17.1 54.7,2 54.1,2.6 v54.1,9.6
  Bottom 0.152: v43.59,65.8 44.09,65.3 44.09,24.28 43.84,24.03 43.84,23.57 44.4,23.01 v44.4,22.9 | v52.7,15.1 54.1,13.7 v54.1,9.6
UP5STLR  (via drill 0.35)
  Top 0.152: v44.4,65.8 42.3,67.9 U1.27 | R16.1 55.3,13.29 52.93,15.66 52.54,15.66 v44.4,23.8
  Bottom 0.152: v44.4,65.8 v44.4,23.8
UP5TX  (via drill 0.35)
  Top 0.152: U1.44 47.2,76.8 v48.4,75.6
  Top 0.203: J1.P$5 60.01,9.4 v60.9,10.3
  Bottom 0.152: v48.4,75.6 53.7,70.3 53.7,69 60.9,61.8 v60.9,10.3
USBDM  (via drill 0.35)
  Top 0.203: U1.45 44.9,77.3 44.7,77.1 v44.7,75.7 | X1.D- 45.95,7.25 J4.P$1
  Bottom 0.203: v44.7,75.7 45.9,74.5 45.9,9.3 J4.P$1
USBDP  (via drill 0.35)
  Top 0.203: U1.46 45.02,77.8 44.88,77.66 44.75,77.66 44.12,77.02 v44.12,76.6 | X1.D+ 46.6,5 46.31,5.29 46.31,7.31 J3.P$1
  Bottom 0.203: J3.P$1 46.26,9.34 46.26,74.65 45.28,75.62 45.28,76.04 44.72,76.6 v44.12,76.6
VDDCORE
  Top 0.203: U1.53 42.8,80.65 arc-90 C6.1 C7.1
VSW
  Top 0.203: C19.2 2.72,75.35 U2.12
  pour Top (no thermals): 2.6,75.5 2.6,73.5 3.4,72.7 9.8,72.7 9.9,72.8 9.9,77.8 8.2,77.8 5.9,75.5
VUSB  (via drill 0.35)
  Top 0.203: U2.3 6.72,76.4 | X1.VBUS v45.3,2.89 v45.3,2.88
  Top 0.305: U2.2 U2.3 6.72,76.39 7.16,76.39 7.6,76.83 7.6,78.7 6.8,79.5 3.4,79.5 2.9,79 v2.9,78.6 | U2.11 2.98,75.85 v2.9,75.93
  Top 0.813: J6.P$1 2.48,64.02 2.48,67.68 1.06,69.11 1.06,71.48 C17.2
  Bottom 0.203: v2.9,75.94 v2.9,75.93 | v45.3,2.88 45.3,2.6
  Bottom 0.305: v2.9,78.6 v2.9,75.94 | v2.9,75.93 2.9,73.32 C17.2
  Bottom 0.813: J6.P$1 2.4,58.9 2.4,33.8 0.9,32.3 0.9,3.9 arc90 3.8,1 43.7,1 45.3,2.6
  other vias: 2.52,72.94

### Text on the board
tPlace: pwr | ticker | usb | packet | error | mkrouter v0.6 | UP0 | reset | traceswo | swclk | swdio | UP1 | UP4 | UP2 | UP3 | UP4 | UP5
bPlace: UP0 | UP1 | usb power < - > external network power | UP2 | big empty spaces / feel like endless durations / until you find it | UP3 | UP4 | UP5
